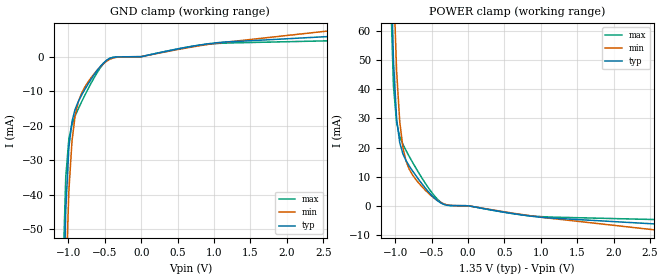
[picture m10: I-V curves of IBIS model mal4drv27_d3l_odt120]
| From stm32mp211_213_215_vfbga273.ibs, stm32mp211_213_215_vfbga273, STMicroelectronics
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[Model] mal4drv27_d3l_odt120
Model_type   Input
Polarity   Non-Inverting
Enable   Active-High
C_comp   1.718pF   1.697pF   1.718pF
C_comp_pullup   843.348fF   826.818fF   845.105fF
C_comp_pulldown   754.530fF   746.726fF   762.427fF
Vinh = 805.000mV
Vinl = 545.000mV
[Model Spec]
D_overshoot_ampl_h 0.4 NA   NA
D_overshoot_ampl_l 0.4 NA   NA
D_overshoot_area_l 110.000m NA   NA
D_overshoot_area_h 110.000m NA   NA
[Temperature Range]   25.000   125.000   -40.000
[Voltage Range]   1.350V   1.283V   1.425V
[GND Clamp Reference]   0.00V   0.00V   0.00V
[C Comp Corner]
| variable   typ   min   max
C_comp   1.718pF   1.697pF   1.718pF
C_comp_pullup   843.348fF   826.818fF   845.105fF
C_comp_pulldown   754.530fF   746.726fF   762.427fF
[POWER Clamp Reference]   1.350V   1.283V   1.425V
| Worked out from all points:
|   GND clamp passes 1 mA (typ) near -0.47 V on its own axis
|   POWER clamp passes 1 mA (typ) near -0.38 V on its own axis
[GND Clamp]
-1.339V   -732mA     -692.4mA   -720.8mA
-1.079V   -84mA      -111.5mA   -66.04mA
-1.036V   -44.58mA   -66.23mA   -34.89mA
-993.2mV  -26.32mA   -38.9mA    -23.83mA
-950mV    -18.76mA   -24.36mA   -19.64mA
-906.8mV  -15.22mA   -17mA      -17.17mA
-863.6mV  -13.02mA   -13.09mA   -15.12mA
-690.9mV  -6.641mA   -6.195mA   -7.798mA
-561.4mV  -2.83mA    -2.928mA   -3.228mA
-431.8mV  -506.4uA   -777.4uA   -471.5uA
950mV     3.822mA    3.657mA    3.685mA
2.677V    5.963mA    7.71mA     4.653mA
[Power Clamp]
-1.327V   872.9mA    828.2mA    856.2mA
-1.068V   93.71mA    131.1mA    76.2mA
-1.025V   49.96mA    78.41mA    41.34mA
-981.8mV  29.98mA    46.45mA    28.58mA
-938.6mV  21.7mA     29.02mA    23.79mA
-895.5mV  17.86mA    20.09mA    21.13mA
-852.3mV  15.54mA    15.38mA    18.99mA
-765.9mV  12.1mA     10.7mA     15.08mA
-679.5mV  9.059mA    7.85mA     11.39mA
-377.3mV  968.7uA    1.128mA    1.249mA
918.2mV   -3.75mA    -3.681mA   -3.597mA
2.689V    -6.443mA   -8.663mA   -4.829mA
